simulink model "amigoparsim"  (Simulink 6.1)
settings: Solver=ode23s  StartTime=0.0  StopTime=400  MaxStep=0.05  RelTol=1e-8
undefined symbols (not defined in the file or in its folder): sys_tf, totaldelay
libraries: simulink x1, cstblocks x1

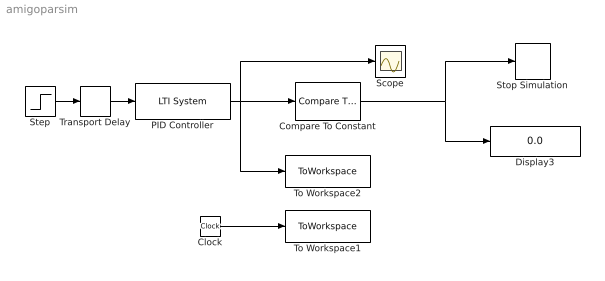
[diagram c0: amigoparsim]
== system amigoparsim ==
  Clock : Clock
  Compare To Constant : simulink/Logic and Bit Operations/Compare To Constant  relop=>=  const=1-exp(-1)  LogicOutDataTypeMode=boolean  ZeroCross=off
  Display3 : Display
  PID Controller : cstblocks/LTI System  sys=syst  IC=[]
  Scope : Scope
  Step : Step  Time=0  SampleTime=0
  Stop Simulation : Stop
  To Workspace1 : ToWorkspace  VariableName=tid  SampleTime=-1  SaveFormat=Array
  To Workspace2 : ToWorkspace  VariableName=step_vals  SampleTime=-1  SaveFormat=Array
  Transport Delay : TransportDelay  DelayTime=totaldelay(sys_tf)  BufferSize=100000
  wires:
  Clock/1 -> To Workspace1/1
  Step/1 -> Transport Delay/1
  PID Controller/1 -> To Workspace2/1, Compare To Constant/1, Scope/1
  Compare To Constant/1 -> Stop Simulation/1, Display3/1
  Transport Delay/1 -> PID Controller/1
